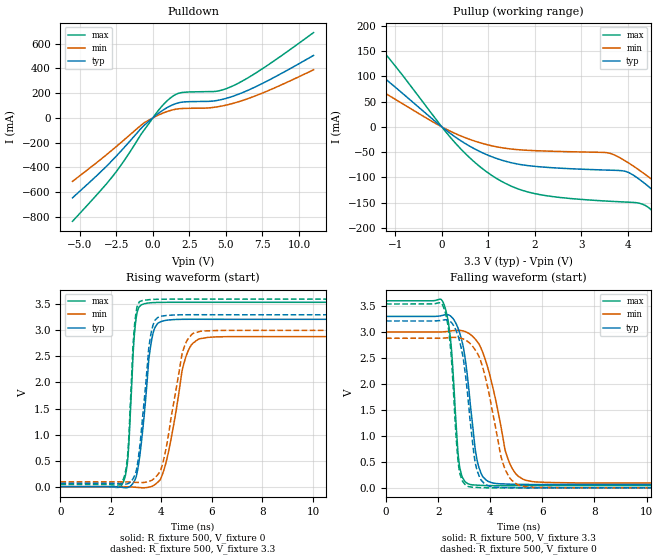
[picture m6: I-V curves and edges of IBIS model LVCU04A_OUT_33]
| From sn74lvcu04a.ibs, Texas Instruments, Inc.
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[Model]   LVCU04A_OUT_33
Model_type  Output
Vref =   0
Rref =   500
Cref =   50p
Vmeas =   1.5
| variable   typ   min   max
C_comp   7.71pF   3.82pF   12.90pF
| C_pullup   6.89pF   3.82pF   8.54pF
| C_pulldown   8.52pF   4.18pF   12.90pF
[Temperature Range]   40   100   -40
| Ambient temperature   25   85   -40
[Voltage range]   3.3   3   3.6
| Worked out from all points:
|   slope of the pulldown table from 0 to 0.495 V, typ, clamps not added: 10.7 ohm
|   slope of the pullup table from 0 to 0.495 V, typ, clamps not added: 15.2 ohm
|   rising waveform, R_fixture 500, V_fixture 0: 20-80 % time 378ps typ, 619ps min, 222ps max; typ from 0 V to 3.21 V
|   falling waveform, R_fixture 500, V_fixture 3.3: 20-80 % time 448ps typ, 761ps min, 283ps max; typ from 3.3 V to 0.065 V
|   rising waveform, R_fixture 500, V_fixture 3.3: 20-80 % time 369ps typ, 613ps min, 217ps max; typ from 0.065 V to 3.3 V
|   falling waveform, R_fixture 500, V_fixture 0: 20-80 % time 440ps typ, 708ps min, 282ps max; typ from 3.21 V to 0 V
[Pulldown]
| LVCU04A_OUT_33
|   Voltage   I(typ)   I(min)   I(max)
-5.5V     -645.8mA   -513mA     -835.8mA
-3.645V   -444.9mA   -342.7mA   -596.4mA
-2.71V    -334.7mA   -252.1mA   -466mA
-1.89V    -230mA     -169.6mA   -332.4mA
-620mV    -62.41mA   -41.52mA   -102.1mA
455mV     42.83mA    26.93mA    71.74mA
1.215V    98.07mA    60.46mA    162.3mA
1.91V     125.9mA    75.23mA    203.5mA
4.31V     139.6mA    87.57mA    214.6mA
5.45V     173.8mA    116.3mA    257.3mA
7.53V     280.4mA    202.4mA    399.9mA
11V       505.3mA    389mA      689.8mA
[Pullup]
| LVCU04A_OUT_33
|   Voltage   I(typ)   I(min)   I(max)
-5.5V     404.4mA    310.8mA    569.2mA
-3.515V   265mA      197.3mA    383.4mA
-2.48V    190.1mA    138.3mA    280.1mA
-1.635V   127.1mA    90.28mA    191.1mA
505mV     -33.05mA   -21.44mA   -52.79mA
1.855V    -76.61mA   -46.34mA   -128.9mA
3.7V      -85.85mA   -55.17mA   -147.6mA
4.24V     -103.4mA   -85.4mA    -151mA
4.89V     -155mA     -131.2mA   -201.1mA
5.36V     -197.9mA   -167.7mA   -253.2mA
5.82V     -242.5mA   -205.2mA   -308.1mA
11V       -792.2mA   -667mA     -979.2mA
[Ramp]
| LVCU04A_OUT_33
| variable   typ   min   max
dV/dt_r   1.94/4.13E-10   1.74/6.80E-10   2.13/2.42E-10
dV/dt_f   1.96/4.65E-10   1.76/8.32E-10   2.15/2.94E-10
R_load = 500
[Rising Waveform]
| LVCU04A_OUT_33
R_fixture =   500
C_fixture =   0
L_fixture =   0
V_fixture =   0
V_fixture_min = 0
V_fixture_max = 0
|   Time   V(typ)   V(min)   V(max)
0s        184.9pV    3.596nV    20.95pV
2.485ns   -15.62mV   230.3uV    85.27mV
2.675ns   -14.72mV   -2.054mV   583.2mV
2.975ns   156.7mV    -11.58mV   3.151V
3.315ns   1.366V     -21.97mV   3.511V
3.755ns   3.066V     45.55mV    3.535V
4.215ns   3.196V     532.2mV    3.539V
4.935ns   3.213V     2.445V     3.54V
5.525ns   3.213V     2.841V     3.54V
24.99ns   3.212V     2.88V      3.539V
[Falling Waveform]
| LVCU04A_OUT_33
R_fixture =   500
C_fixture =   0
L_fixture =   0
V_fixture =   3.3
V_fixture_min = 3
V_fixture_max = 3.6
|   Time   V(typ)   V(min)   V(max)
0s        3.3V       3V         3.6V
2.2ns     3.324V     3.003V     3.56V
2.495ns   3.299V     3.021V     2.755V
2.81ns    3.007V     3.031V     456.9mV
3.18ns    1.887V     2.972V     71.24mV
3.435ns   701.4mV    2.856V     53.65mV
3.7ns     225.6mV    2.621V     46.04mV
4.645ns   72.16mV    606.6mV    41.04mV
5.36ns    64.58mV    145.8mV    41.62mV
24.99ns   64.52mV    92.1mV     41.93mV
[Rising Waveform]
| LVCU04A_OUT_33
R_fixture =   500
C_fixture =   0
L_fixture =   0
V_fixture =   3.3
V_fixture_min = 3
V_fixture_max = 3.6
|   Time   V(typ)   V(min)   V(max)
0s        64.52mV    92.1mV     41.93mV
2.48ns    52.91mV    92.24mV    134.2mV
2.665ns   57.16mV    90.24mV    633.1mV
2.935ns   213.6mV    83.78mV    3.106V
3.155ns   836.6mV    79.73mV    3.561V
3.71ns    3.161V     157.4mV    3.596V
4.115ns   3.28V      578mV      3.599V
4.825ns   3.3V       2.563V     3.6V
5.33ns    3.301V     2.962V     3.6V
24.99ns   3.3V       3V         3.6V
[Falling Waveform]
| LVCU04A_OUT_33
R_fixture =   500
C_fixture =   0
L_fixture =   0
V_fixture =   0
V_fixture_min = 0
V_fixture_max = 0
|   Time   V(typ)   V(min)   V(max)
0s        3.212V     2.88V      3.539V
2.19ns    3.231V     2.882V     3.497V
2.455ns   3.207V     2.893V     2.796V
2.795ns   2.876V     2.888V     384.8mV
3.175ns   1.57V      2.801V     22.59mV
3.395ns   569.5mV    2.675V     9.339mV
3.635ns   158.5mV    2.439V     4.182mV
4.48ns    5.997mV    484.9mV    -680.8uV
5.14ns    300.5uV    44.99mV    -361.3uV
24.99ns   14.56nV    13.22nV    249.9pV
